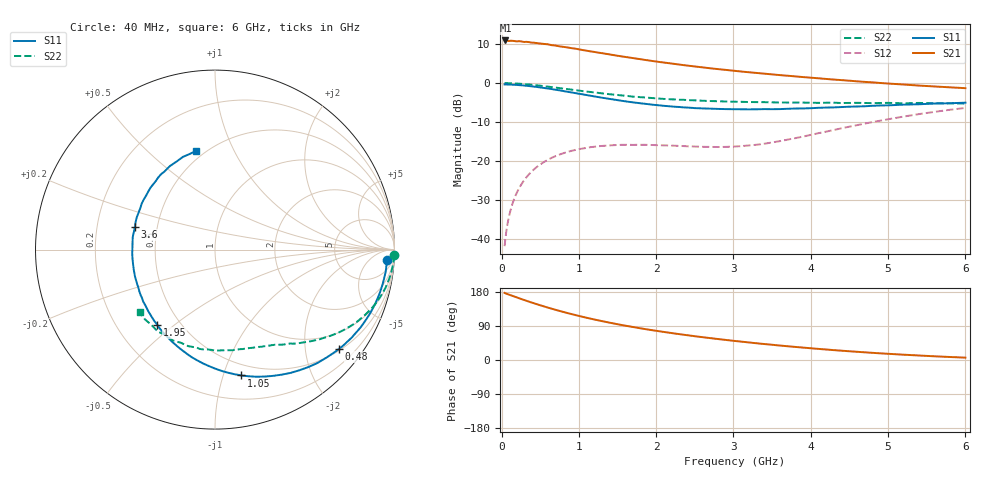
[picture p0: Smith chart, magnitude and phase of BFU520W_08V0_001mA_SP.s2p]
! Filename:  P:\Prog\Test\Noise\ATS_data\Testdata_Net\Run2\BFU520W_APM2013_06_A05_08p0V_001mA_SP_CM01_D.s2p
! Date/Time: Tue 26/Mar/2013 18:01:41
! BFU520W_APM2013_06_A05_08p0V_1to20mA_SP_CM01_Bias1_R.s2p
! MDIF S-parameter v. bias file
! BFU520W_APM2013_06_A05_08p0V_1to20mA_SP_CM01
! Date/time Thu Mar 21 15:28:29 2013
! bias mode 1
! bias variable = I_out
! VAR bias_var= 1
! VAR V_out= 8.0000
! VAR I_out= 1.0000
! VAR V_in= 0.7917
! VAR I_in= 0.0107
! Device data file deembeded for feedlines and parallel
! Original file: \Run2\BFU520W_APM2013_06_A05_08p0V_001mA_SP_CM01_R.s2p
! Feed-files: PR019V01_070313_Feed1.s2p, PR019V01_070313_Feed2.s2p
! Parallel-file: PR019V01_070313_Par.s2p
# MHz S MA R 50
!  Freq-MHz  S11-mag  S11-arg  S21-mag  S21-arg  S12-mag  S12-arg  S22-mag  S22-arg
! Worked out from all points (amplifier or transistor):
!   98 points, 40 MHz to 6 GHz, reference 50 ohm
!   highest |S21| = 10.9 dB at 50 MHz (marker M1)
!   |S21| within 3 dB of that: start of sweep to 1.217 GHz
!   unconditionally stable (mu >= 1): 2.774 GHz to 3.73 GHz
!   at 300 MHz: K = 0.12, MSG = 17.6 dB, |S12| = -24.7 dB
!   at 1.6 GHz: K = 0.57, MSG = 11.3 dB, |S12| = -15.8 dB
!   at 6 GHz: K = 0.80, MSG = 2.5 dB, |S12| = -6.4 dB
!   S11 on the Smith chart (normalised r, x): 40 MHz: 16, -23; 480 MHz: 0.54, -2.75; 1.05 GHz: 0.40, -1.15; 1.95 GHz: 0.38, -0.44; 3.6 GHz: 0.37, +0.12; 6 GHz: 0.45, +0.72
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40  0.9602 -3.3  3.502 177.1  0.008121 87.5  0.9982 -1.8
50  0.9606 -4.2  3.516 176.0  0.0101 87.2  0.9987 -2.2
100  0.9575 -8.3  3.462 172.3  0.02017 84.3  0.995 -4.7
120  0.9555 -10.0  3.49 170.8  0.02414 83.2  0.9941 -5.5
200  0.9461 -16.5  3.422 165.0  0.03973 78.9  0.985 -9.2
240  0.9393 -19.9  3.438 162.0  0.04722 76.9  0.9794 -11.0
340  0.9202 -27.9  3.364 155.1  0.06505 71.8  0.9609 -15.3
480  0.8849 -38.7  3.221 145.8  0.08757 65.3  0.9307 -20.8
600  0.8516 -47.9  3.139 138.3  0.1041 60.1  0.9002 -25.1
700  0.8206 -55.0  3.026 132.3  0.1159 56.2  0.8748 -28.5
850  0.7744 -65.3  2.864 124.0  0.1307 51.0  0.8371 -33.0
1050  0.7163 -78.2  2.65 113.9  0.1449 45.1  0.7884 -38.2
1250  0.662 -90.2  2.456 104.7  0.155 40.3  0.7486 -42.6
1500  0.6045 -104.3  2.24 94.4  0.1609 35.6  0.7033 -47.7
1950  0.5279 -127.5  1.918 78.6  0.1608 31.4  0.6429 -55.5
2050  0.5172 -132.3  1.859 75.6  0.1595 31.3  0.6318 -57.0
2500  0.4776 -153.1  1.633 62.8  0.1537 33.1  0.6007 -64.3
3100  0.4615 -177.8  1.406 48.5  0.1555 44.2  0.5751 -74.5
3600  0.4637 164.2  1.265 38.2  0.1802 54.5  0.5639 -83.9
4100  0.4818 148.1  1.152 29.3  0.228 60.0  0.5575 -94.3
5200  0.529 118.3  0.9581 14.0  0.3721 56.1  0.5501 -119.7
6000  0.5607 100.7  0.8604 6.2  0.4801 46.9  0.5455 -140.4
